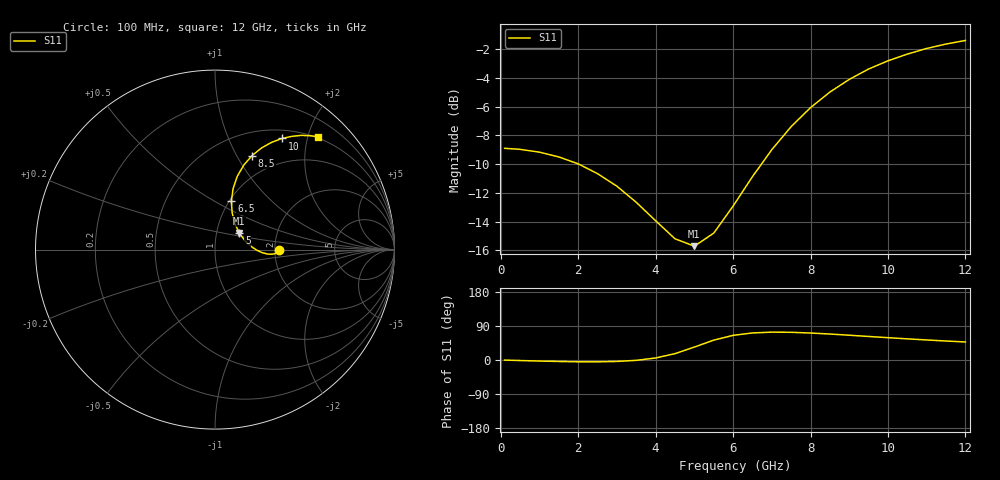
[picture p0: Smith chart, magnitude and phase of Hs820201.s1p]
!HSMS-8101 and HSMS-8202 Schottky diodes
!S-parameters at 1 mA self-bias.  Last updated 6/7/94
# ghz s ma r 50
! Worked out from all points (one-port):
!   25 points, 100 MHz to 12 GHz, reference 50 ohm
!   lowest |S11| = -15.7 dB at 5 GHz (marker M1), VSWR 1.39, Z = 64.4 + j12.2 ohm
!   |S11| at or under -10 dB: 2.015 GHz to 6.732 GHz (4.717 GHz wide, 108 % of centre)
!   S11 on the Smith chart (normalised r, x): 100 MHz: 2.12, -0.01; 5 GHz: 1.29, +0.24; 6.5 GHz: 1.02, +0.60; 8.5 GHz: 0.76, +1.16; 10 GHz: 0.62, +1.60; 12 GHz: 0.48, +2.18
0.1  0.359 -0.3
0.5  0.356 -1.4
1  0.348 -2.8
1.5  0.335 -3.9
2  0.317 -4.7
2.5  0.293 -4.8
3  0.265 -3.8
3.5  0.233 -0.9
4  0.201 5.3
4.5  0.174 16.8
5  0.164 34.1
5.5  0.182 52.4
6  0.226 65.0
6.5  0.286 71.4
7  0.355 73.5
7.5  0.427 73.1
8  0.497 71.2
8.5  0.563 68.5
9  0.623 65.4
9.5  0.677 62.1
10  0.723 58.9
10.5  0.763 55.8
11  0.798 52.9
11.5  0.827 50.1
12  0.851 47.6
